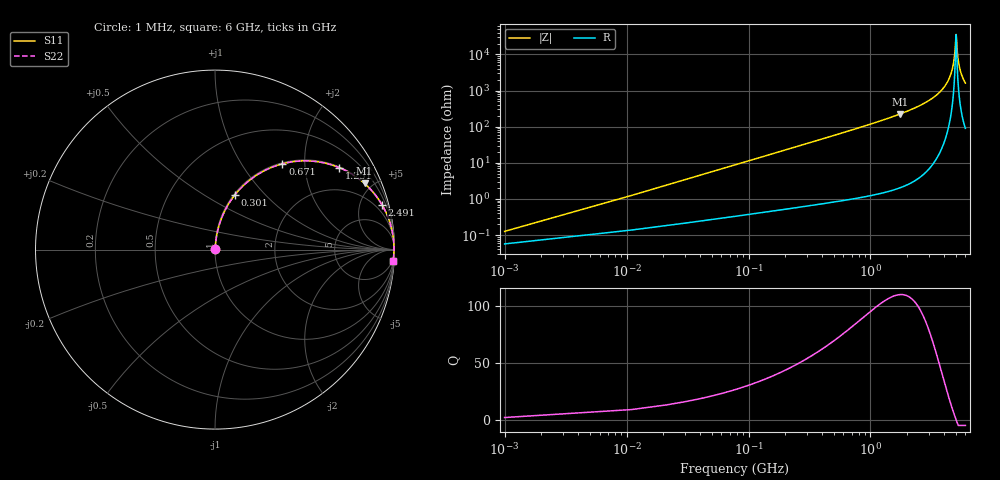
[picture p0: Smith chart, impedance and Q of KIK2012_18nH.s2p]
!version-2
!date-01.2022
!Series
# MHz S RI R 50
!Freq ReS11 ImS11 ReS21 ImS21 ReS12 ImS12 ReS22 ImS22
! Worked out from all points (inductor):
!   601 points, 1 MHz to 6 GHz, reference 50 ohm
!   read as one part in series: L = 18 nH near 31 MHz
!   highest Q = 110 at 1.751 GHz (marker M1), where L = 20.5 nH
!   self-resonance near 5.031 GHz
!   S11 on the Smith chart (normalised r, x): 1 MHz: 1.00, +0.00; 301 MHz: 1.01, +0.68; 671 MHz: 1.02, +1.55; 1.251 GHz: 1.03, +3.02; 2.491 GHz: 1.08, +7.46; 6 GHz: 3, -32
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1  0.00057 0.00113  0.9994 -0.00113  0.9994 -0.00113  0.00057 0.00113
41  0.00458 0.046  0.9954 -0.046  0.9954 -0.046  0.00458 0.046
71  0.00951 0.0793  0.9905 -0.0793  0.9905 -0.0793  0.00951 0.0793
161  0.0364 0.1748  0.9636 -0.1748  0.9636 -0.1748  0.0364 0.1748
301  0.109 0.3025  0.891 -0.3025  0.891 -0.3025  0.109 0.3025
671  0.3753 0.478  0.6247 -0.478  0.6247 -0.478  0.3753 0.478
1001  0.5807 0.4882  0.4193 -0.4882  0.4193 -0.4882  0.5807 0.4882
1251  0.6928 0.4565  0.3072 -0.4565  0.3072 -0.4565  0.6928 0.4565
1751  0.8331 0.3683  0.1669 -0.3683  0.1669 -0.3683  0.8331 0.3683
2001  0.8761 0.3249  0.1239 -0.3249  0.1239 -0.3249  0.8761 0.3249
2491  0.9308 0.2489  0.0692 -0.2489  0.0692 -0.2489  0.9308 0.2489
3001  0.963 0.1825  0.037 -0.1825  0.037 -0.1825  0.963 0.1825
4001  0.9911 0.0806  0.0089 -0.0806  0.0089 -0.0806  0.9911 0.0806
4411  0.9954 0.0463  0.00463 -0.0463  0.00463 -0.0463  0.9954 0.0463
4701  0.9968 0.024  0.00318 -0.024  0.00318 -0.024  0.9968 0.024
4881  0.9972 0.0109  0.00281 -0.0109  0.00281 -0.0109  0.9972 0.0109
5001  0.9972 0.00244  0.00276 -0.00244  0.00276 -0.00244  0.9972 0.00244
5051  0.9972 -0.00104  0.00278 0.00104  0.00278 0.00104  0.9972 -0.00104
5191  0.997 -0.0106  0.00298 0.0106  0.00298 0.0106  0.997 -0.0106
5381  0.9965 -0.0231  0.00352 0.0231  0.00352 0.0231  0.9965 -0.0231
5641  0.9953 -0.0396  0.00474 0.0396  0.00474 0.0396  0.9953 -0.0396
6000  0.9928 -0.0611  0.0072 0.0611  0.0072 0.0611  0.9928 -0.0611
